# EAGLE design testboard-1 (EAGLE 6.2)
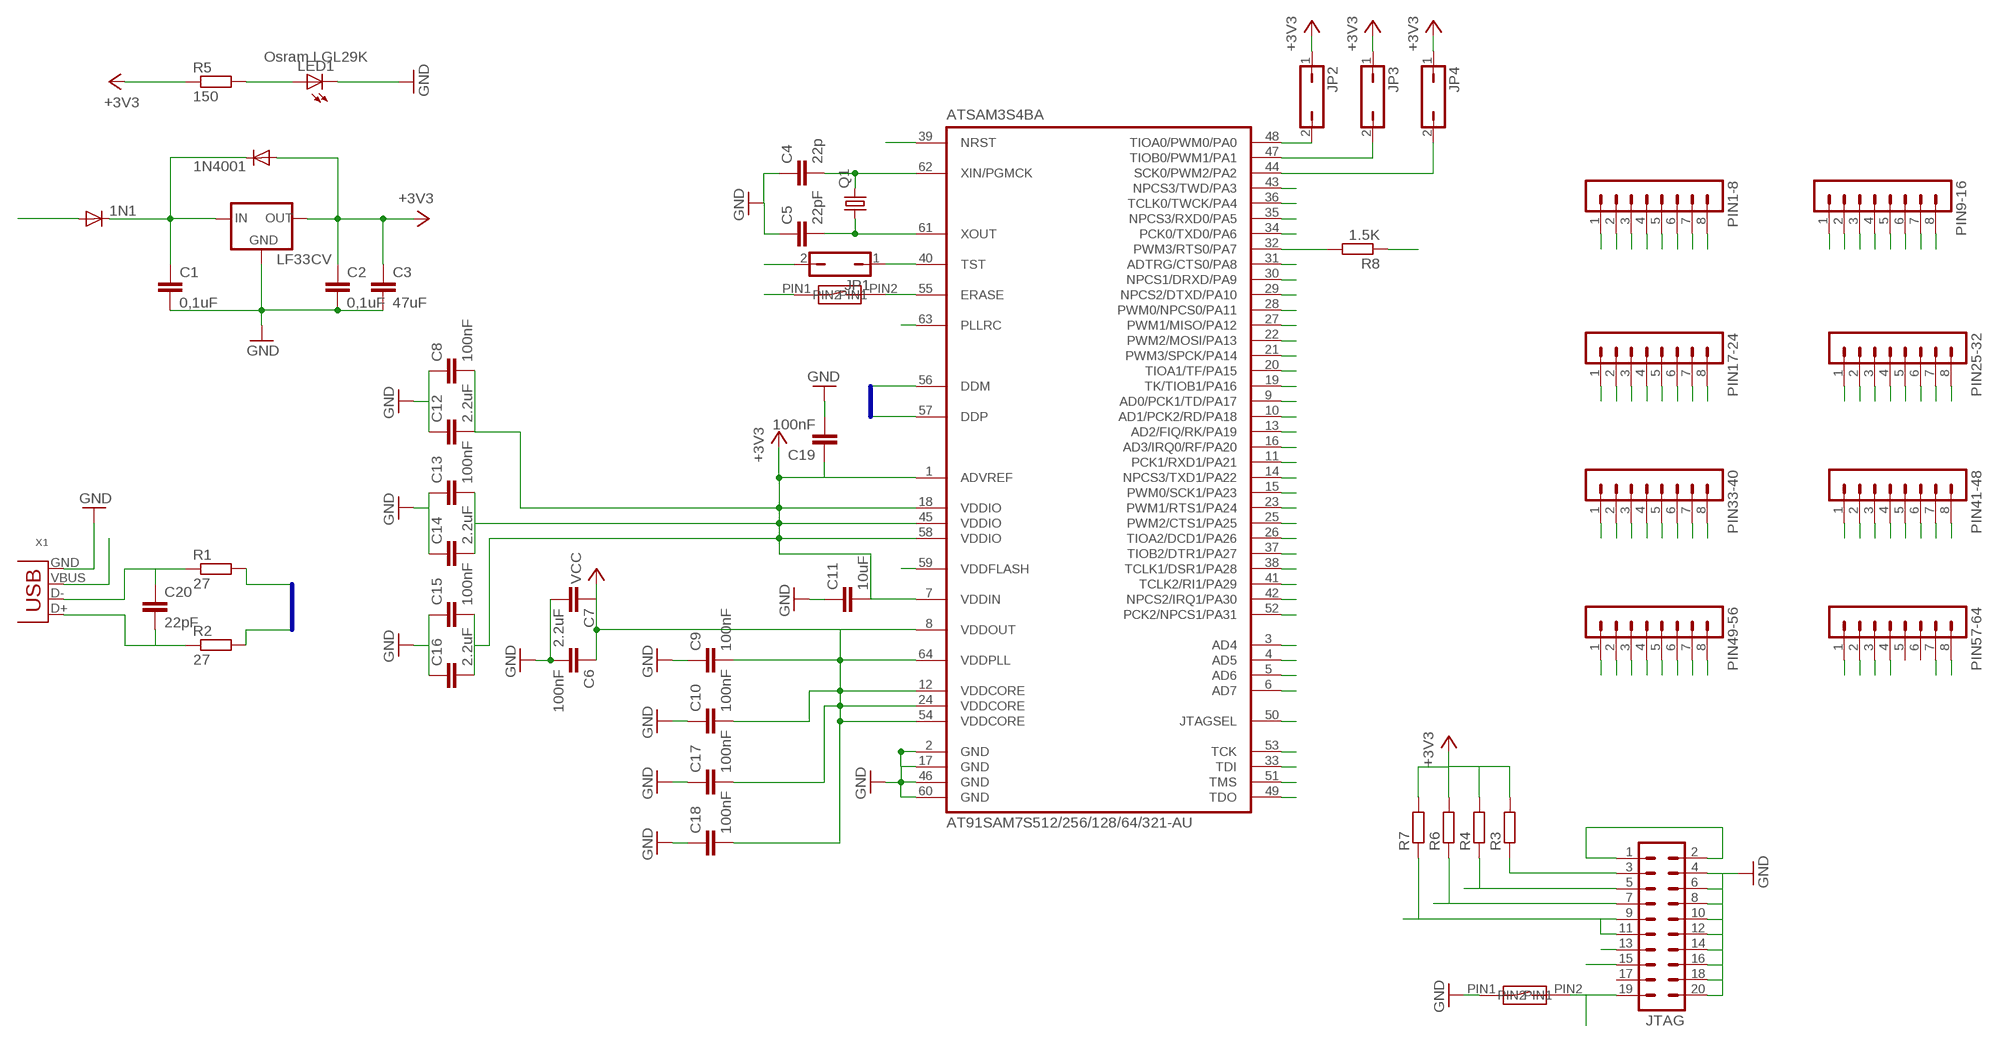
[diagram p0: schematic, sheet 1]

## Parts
1N1  DIODE-MELF-MLL41  [MELF-MLL41]
1N4001  DIODE-MELF-MLL41  [MELF-MLL41]
ATSAM3S4BA  AT91SAM7S512/256/128/64/321-AU  [LQFP64]
C1  0,1uF  C-EUC0805  [C0805]
C2  0,1uF  C-EUC0805  [C0805]
C3  47uF  C-EUC1206  [C1206]
C4  22p  C-EUC0805  [C0805]
C5  22pF  C-EUC0805  [C0805]
C6  100nF  C-EUC0603  [C0603]
C7  2.2uF  C-EUC0603  [C0603]
C8  100nF  C-EUC0603  [C0603]
C9  100nF  C-EUC0603K  [C0603K]
C10  100nF  C-EUC0603  [C0603]
C11  10uF  C-EUC0603  [C0603]
C12  2.2uF  C-EUC0603  [C0603]
C13  100nF  C-EUC0603  [C0603]
C14  2.2uF  C-EUC0603  [C0603]
C15  100nF  C-EUC0603  [C0603]
C16  2.2uF  C-EUC0603  [C0603]
C17  100nF  C-EUC0603  [C0603]
C18  100nF  C-EUC0603  [C0603]
C19  100nF  C-EUC0603  [C0603]
C20  22pF  C-EUC0603  [C0603]
JP1  JP1Q  [JP1]
JP2  JP1Q  [JP1]
JP3  JP1Q  [JP1]
JP4  JP1Q  [JP1]
JTAG  MA10-2  [MA10-2]
LED1  LEDSML0603  [SML0603]
LF33CV  78XXL  [78XXL]
PIN1-8  MA08-1  [MA08-1]
PIN9-16  MA08-1  [MA08-1]
PIN17-24  MA08-1  [MA08-1]
PIN25-32  MA08-1  [MA08-1]
PIN33-40  MA08-1  [MA08-1]
PIN41-48  MA08-1  [MA08-1]
PIN49-56  MA08-1  [MA08-1]
PIN57-64  MA08-1  [MA08-1]
Q1  CRYSTALHC49S  [HC49/S]
R1  27  R-EU_R0603  [R0603]
R2  27  R-EU_R0603  [R0603]
R3  R-EU_R0603  [R0603]
R4  R-EU_R0603  [R0603]
R5  150  R-EU_M0805  [M0805]
R6  R-EU_R0603  [R0603]
R7  R-EU_R0603  [R0603]
R8  1.5K  R-EU_R0603  [R0603]
SWITCH1  SDT21S  [DIL-2]
SWITCH2  SDT21S  [DIL-2]
X1  USB-B-H  [USB-B-H]

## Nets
+3V3: 1N4001.A ATSAM3S4BA.1(ADVREF) ATSAM3S4BA.7(VDDIN) ATSAM3S4BA.18(VDDIO) ATSAM3S4BA.45(VDDIO) ATSAM3S4BA.58(VDDIO) C2.1 C3.1 C8.2 C11.2 C12.2 C13.2 C14.2 C15.2 C16.2 C19.1 JP2.1 JP3.1 JP4.1 LF33CV.OUT R3.2 R4.2 R5.1 R6.2 R7.2
GND: ATSAM3S4BA.2(GND) ATSAM3S4BA.17(GND) ATSAM3S4BA.46(GND) ATSAM3S4BA.60(GND) C1.2 C2.2 C3.2 C4.1 C5.1 C6.2 C7.2 C8.1 C9.1 C10.1 C11.1 C12.1 C13.1 C14.1 C15.1 C16.1 C17.1 C18.1 C19.2 JTAG.4 JTAG.6 JTAG.8 JTAG.10 JTAG.12 JTAG.14 JTAG.16 JTAG.18 JTAG.20 LED1.C LF33CV.GND SWITCH2.PIN1 X1.GND
N$7: C20.1 R1.1 X1.D-
N$13: LED1.A R5.2
N$14: ATSAM3S4BA.59(VDDFLASH)
N$15: ATSAM3S4BA.55(ERASE) SWITCH1.PIN2
N$18: JTAG.3 R3.1
NRST: ATSAM3S4BA.39(NRST) JTAG.15 JTAG.19 SWITCH2.PIN2
PIN1: PIN1-8.1
PIN2: PIN1-8.2
PIN3: ATSAM3S4BA.3(AD4) PIN1-8.3
PIN4: ATSAM3S4BA.4(AD5) PIN1-8.4
PIN5: ATSAM3S4BA.5(AD6) PIN1-8.5
PIN6: ATSAM3S4BA.6(AD7) PIN1-8.6
PIN7: PIN1-8.7
PIN8: PIN1-8.8
PIN9: ATSAM3S4BA.9(AD0/PCK1/TD/PA17) PIN9-16.1
PIN10: ATSAM3S4BA.10(AD1/PCK2/RD/PA18) PIN9-16.2
PIN11: ATSAM3S4BA.11(PCK1/RXD1/PA21) PIN9-16.3
PIN12: PIN9-16.4
PIN13: ATSAM3S4BA.13(AD2/FIQ/RK/PA19) PIN9-16.5
PIN14: ATSAM3S4BA.14(NPCS3/TXD1/PA22) PIN9-16.6
PIN15: ATSAM3S4BA.15(PWM0/SCK1/PA23) PIN9-16.7
PIN16: ATSAM3S4BA.16(AD3/IRQ0/RF/PA20) PIN9-16.8
PIN17: PIN17-24.1
PIN18: PIN17-24.2
PIN19: ATSAM3S4BA.19(TK/TIOB1/PA16) PIN17-24.3
PIN20: ATSAM3S4BA.20(TIOA1/TF/PA15) PIN17-24.4
PIN21: ATSAM3S4BA.21(PWM3/SPCK/PA14) PIN17-24.5
PIN22: ATSAM3S4BA.22(PWM2/MOSI/PA13) PIN17-24.6
PIN23: ATSAM3S4BA.23(PWM1/RTS1/PA24) PIN17-24.7
PIN24: PIN17-24.8
PIN25: ATSAM3S4BA.25(PWM2/CTS1/PA25) PIN25-32.1
PIN26: ATSAM3S4BA.26(TIOA2/DCD1/PA26) PIN25-32.2
PIN27: ATSAM3S4BA.27(PWM1/MISO/PA12) PIN25-32.3
PIN28: ATSAM3S4BA.28(PWM0/NPCS0/PA11) PIN25-32.4
PIN29: ATSAM3S4BA.29(NPCS2/DTXD/PA10) PIN25-32.5
PIN30: ATSAM3S4BA.30(NPCS1/DRXD/PA9) PIN25-32.6
PIN31: ATSAM3S4BA.31(ADTRG/CTS0/PA8) PIN25-32.7
PIN32: ATSAM3S4BA.32(PWM3/RTS0/PA7) PIN25-32.8 R8.2
PIN33: ATSAM3S4BA.33(TDI) JTAG.5 PIN33-40.1 R4.1
PIN34: ATSAM3S4BA.34(PCK0/TXD0/PA6) PIN33-40.2
PIN35: ATSAM3S4BA.35(NPCS3/RXD0/PA5) PIN33-40.3
PIN36: ATSAM3S4BA.36(TCLK0/TWCK/PA4) PIN33-40.4
PIN37: ATSAM3S4BA.37(TIOB2/DTR1/PA27) PIN33-40.5
PIN38: ATSAM3S4BA.38(TCLK1/DSR1/PA28) PIN33-40.6
PIN39: PIN33-40.7
PIN40: ATSAM3S4BA.40(TST) JP1.1 PIN33-40.8
PIN41: ATSAM3S4BA.41(TCLK2/RI1/PA29) PIN41-48.1
PIN42: ATSAM3S4BA.42(NPCS2/IRQ1/PA30) PIN41-48.2
PIN43: ATSAM3S4BA.43(NPCS3/TWD/PA3) PIN41-48.3
PIN44: ATSAM3S4BA.44(SCK0/PWM2/PA2) JP4.2 PIN41-48.4
PIN45: PIN41-48.5
PIN46: PIN41-48.6
PIN47: ATSAM3S4BA.47(TIOB0/PWM1/PA1) JP3.2 PIN41-48.7
PIN48: ATSAM3S4BA.48(TIOA0/PWM0/PA0) JP2.2 PIN41-48.8
PIN49: ATSAM3S4BA.49(TDO) JTAG.13 PIN49-56.1
PIN50: ATSAM3S4BA.50(JTAGSEL) PIN49-56.2
PIN51: ATSAM3S4BA.51(TMS) JTAG.7 PIN49-56.3 R6.1
PIN52: ATSAM3S4BA.52(PCK2/NPCS1/PA31) PIN49-56.4
PIN53: ATSAM3S4BA.53(TCK) JTAG.9 JTAG.11 PIN49-56.5 R7.1
PIN54: PIN49-56.6
PIN55: PIN49-56.7
PIN56: PIN49-56.8
PIN57: PIN57-64.1
PIN58: PIN57-64.2
PIN59: PIN57-64.3
PIN60: PIN57-64.4
PIN61: ATSAM3S4BA.61(XOUT) C5.2 Q1.1
PIN62: ATSAM3S4BA.62(XIN/PGMCK) C4.2 Q1.2
PIN63: ATSAM3S4BA.63(PLLRC) PIN57-64.7
PIN64: PIN57-64.8
USB_5V: 1N1.A X1.VBUS
USB_MINUS: ATSAM3S4BA.56(DDM) R1.2
USB_PLUS: ATSAM3S4BA.57(DDP) R2.2
USB_PLUS_GEHAUSE: C20.2 R2.1 R8.1 X1.D+
VCC18: ATSAM3S4BA.8(VDDOUT) ATSAM3S4BA.12(VDDCORE) ATSAM3S4BA.24(VDDCORE) ATSAM3S4BA.54(VDDCORE) ATSAM3S4BA.64(VDDPLL) C6.1 C7.1 C9.2 C10.2 C17.2 C18.2 JP1.2 JTAG.1 JTAG.2 SWITCH1.PIN1 ; supply symbol labelled VCC
VX: 1N1.C 1N4001.C C1.1 LF33CV.IN
Unconnected: JTAG.17 PIN57-64.5 PIN57-64.6

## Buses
B$2
B$1

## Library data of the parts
1N1 1N4001 = diode:DIODE-: DIODE
ATSAM3S4BA = atmel-arm:AT91SAM7S512/256/128/64/321: AT91SAM7S512/256/128/64/321 ARM7 Processor
C1-C20 = rcl:C-EU: CAPACITOR, European symbol
JP1-JP4 = jumper:JP1Q: JUMPER
JTAG = con-lstb:MA10-2: PIN HEADER; OC_FARNELL: unknown; OC_NEWARK: unknown
LED1 = led:LED: LED; PRODUCT: Osram LGL29K
LF33CV = v-reg:78XXL: VOLTAGE REGULATOR
PIN1-8 PIN9-16 PIN17-24 PIN25-32 PIN33-40 PIN41-48 PIN49-56 PIN57-64 = con-lstb:MA08-1: PIN HEADER; OC_FARNELL: unknown; OC_NEWARK: unknown
Q1 = crystal:CRYSTAL: CRYSTAL; OC_FARNELL: 1667008; OC_NEWARK: unknown
R1-R8 = rcl:R-EU_: RESISTOR, European symbol
SWITCH1 SWITCH2 = reichelt:SDT21S: "Reichelt Switch - 2 DIL"
X1 = con-usb-3:USB: USB Connectors

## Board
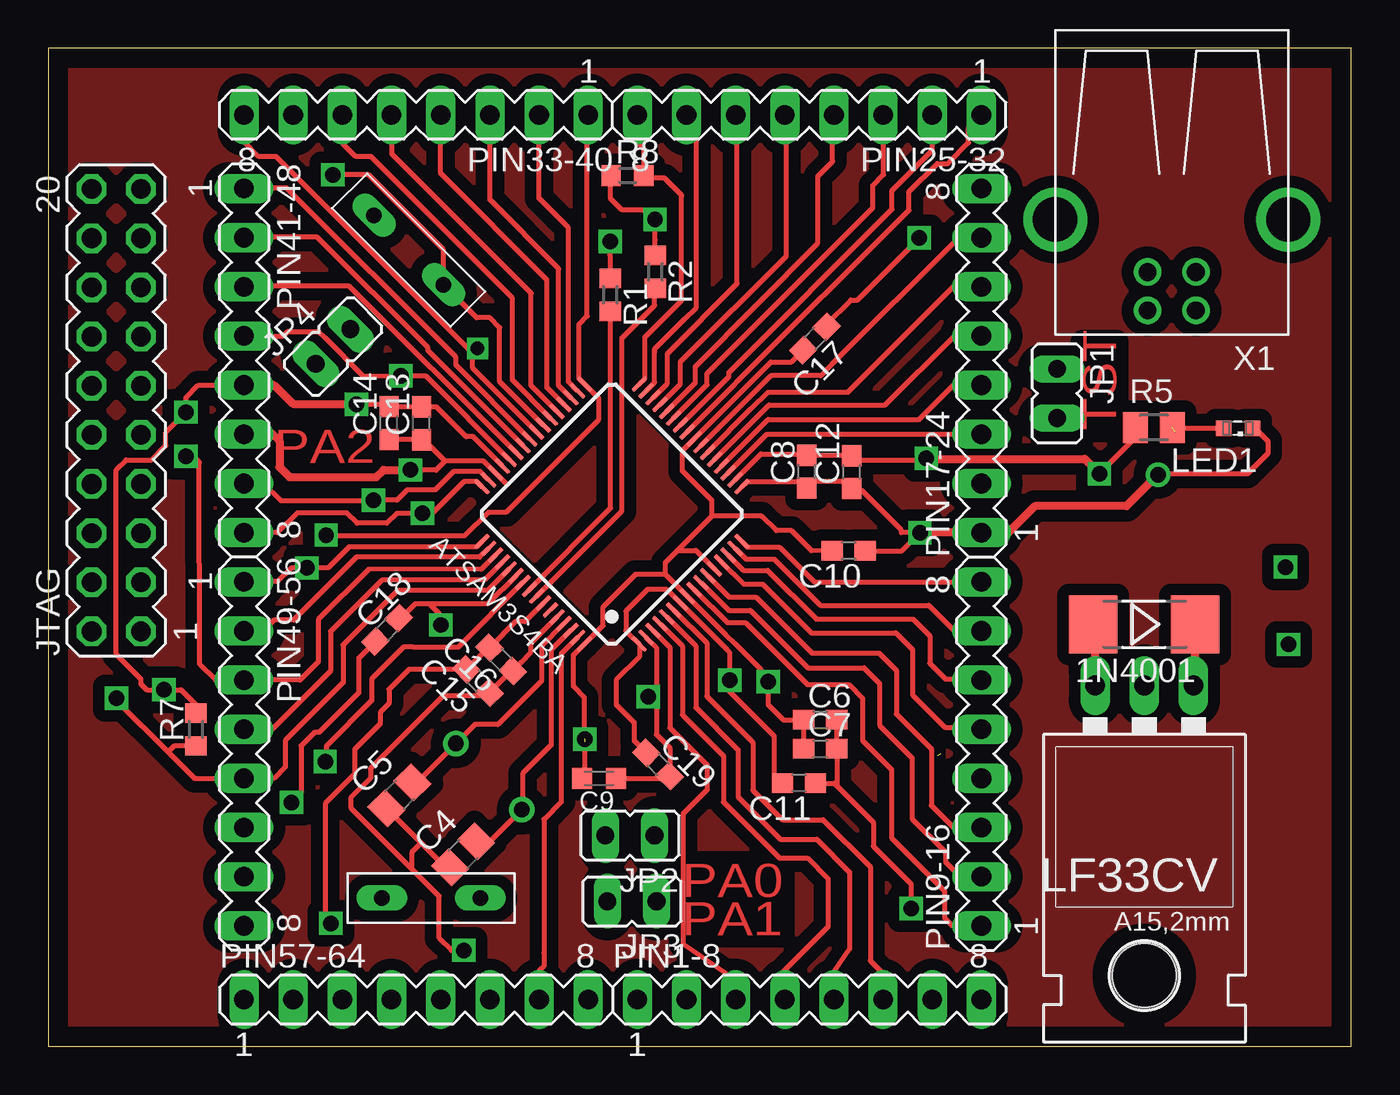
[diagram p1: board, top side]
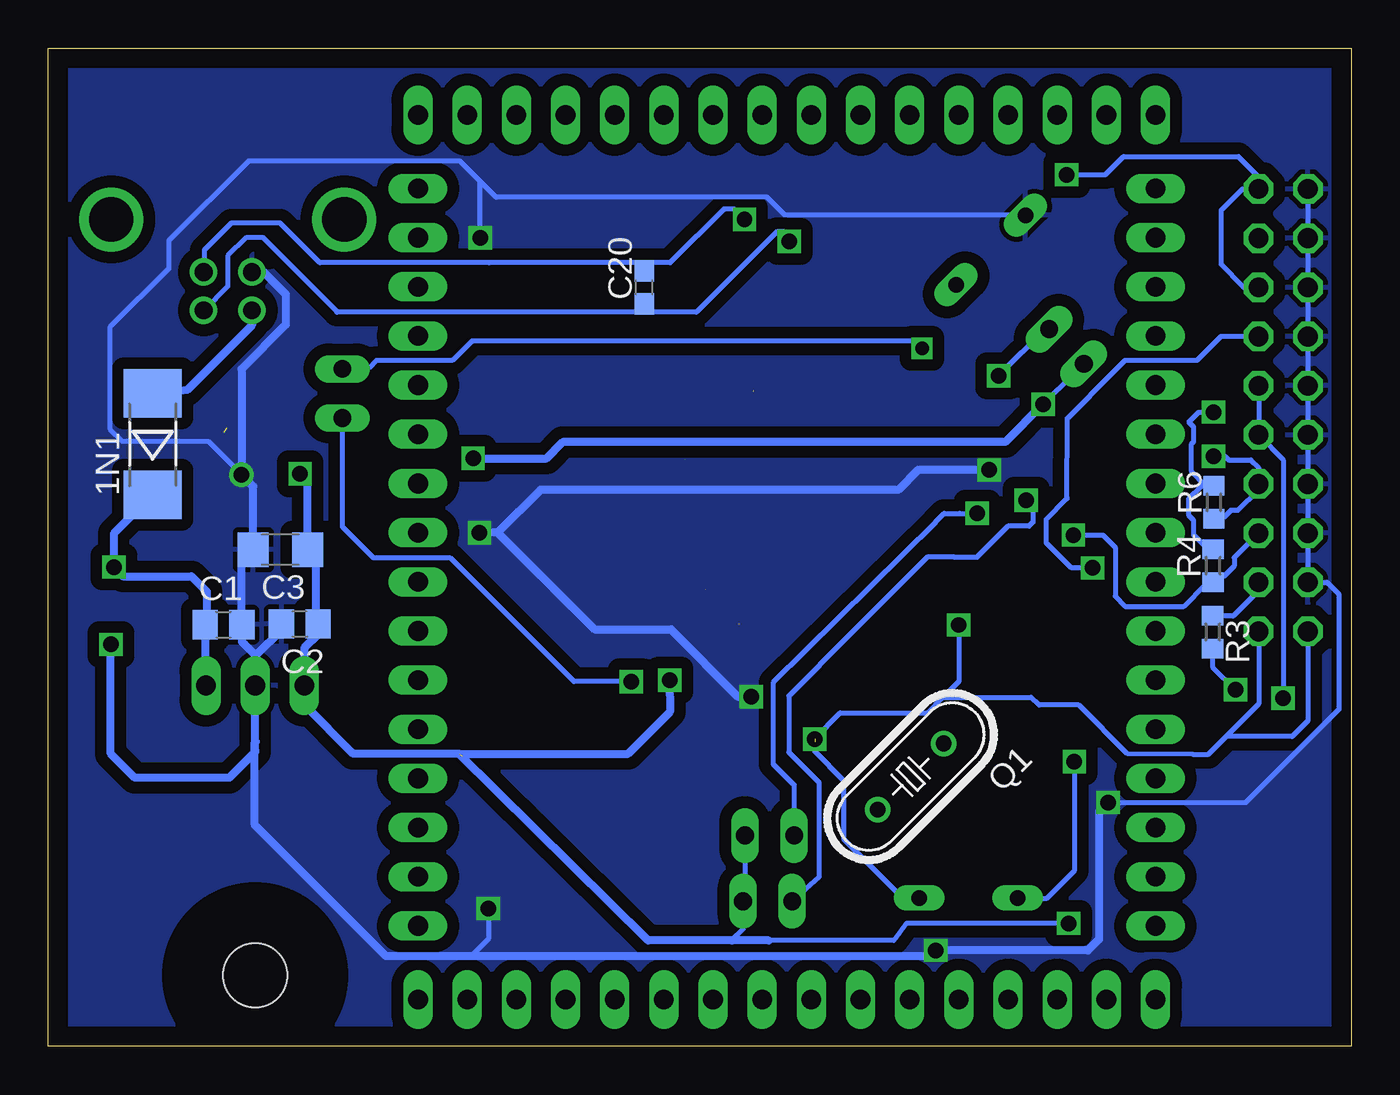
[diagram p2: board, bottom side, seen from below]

Size 67.31 x 51.56 mm. Coordinates in mm from the lower left corner, seen from the top.
Outline: 0,0 67.31,0 67.31,51.56 0,51.56 0,0
Copper layers (1*16): Top 0.035mm / dielectric 1.5mm / Bottom 0.035mm
Design rules "default": minimum track width 10mil, minimum drill 24mil, track to track 8mil, track to pad 8mil, pad to pad 8mil, via to via 8mil, smd to smd 8mil, copper to edge 40mil, drill to drill 8mil, minimum pad ring 10mil, minimum via ring 8mil, stop-mask expansion 4mil, vias tented up to drill 0mil, thermal gap 10mil

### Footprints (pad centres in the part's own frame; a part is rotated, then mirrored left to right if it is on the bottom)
MELF-MLL41 = smd 2.5 x 3: A 2.625,0; C -2.625,0
LQFP64 = smd 0.25 x 1: 1 -3.75,-5.75; 2 -3.25,-5.75; 3 -2.75,-5.75; 4 -2.25,-5.75; 5 -1.75,-5.75; 6 -1.25,-5.75; 7 -0.75,-5.75; 8 -0.25,-5.75; 9 0.25,-5.75; 10 0.75,-5.75; 11 1.25,-5.75; 12 1.75,-5.75; 13 2.25,-5.75; 14 2.75,-5.75; 15 3.25,-5.75; 16 3.75,-5.75; 33 3.75,5.75; 34 3.25,5.75; 35 2.75,5.75; 36 2.25,5.75; 37 1.75,5.75; 38 1.25,5.75; 39 0.75,5.75; 40 0.25,5.75; 41 -0.25,5.75; 42 -0.75,5.75; 43 -1.25,5.75; 44 -1.75,5.75; 45 -2.25,5.75; 46 -2.75,5.75; 47 -3.25,5.75; 48 -3.75,5.75 | smd 1 x 0.25: 17 5.75,-3.75; 18 5.75,-3.25; 19 5.75,-2.75; 20 5.75,-2.25; 21 5.75,-1.75; 22 5.75,-1.25; 23 5.75,-0.75; 24 5.75,-0.25; 25 5.75,0.25; 26 5.75,0.75; 27 5.75,1.25; 28 5.75,1.75; 29 5.75,2.25; 30 5.75,2.75; 31 5.75,3.25; 32 5.75,3.75; 49 -5.75,3.75; 50 -5.75,3.25; 51 -5.75,2.75; 52 -5.75,2.25; 53 -5.75,1.75; 54 -5.75,1.25; 55 -5.75,0.75; 56 -5.75,0.25; 57 -5.75,-0.25; 58 -5.75,-0.75; 59 -5.75,-1.25; 60 -5.75,-1.75; 61 -5.75,-2.25; 62 -5.75,-2.75; 63 -5.75,-3.25; 64 -5.75,-3.75
C0805 = smd 1.3 x 1.5: 1 -0.95,0; 2 0.95,0
C1206 = smd 1.6 x 1.8: 1 -1.4,0; 2 1.4,0
C0603 = smd 1.1 x 1: 1 -0.85,0; 2 0.85,0
C0603K = smd 1.05 x 1.08: 1 -0.875,0; 2 0.875,0
JP1 = drill 0.914 long: 1 0,-1.27; 2 0,1.27
MA10-2 = drill 1.016 octagon: 1 -11.43,-1.27; 2 -11.43,1.27; 3 -8.89,-1.27; 4 -8.89,1.27; 5 -6.35,-1.27; 6 -6.35,1.27; 7 -3.81,-1.27; 8 -3.81,1.27; 9 -1.27,-1.27; 10 -1.27,1.27; 11 1.27,-1.27; 12 1.27,1.27; 13 3.81,-1.27; 14 3.81,1.27; 15 6.35,-1.27; 16 6.35,1.27; 17 8.89,-1.27; 18 8.89,1.27; 19 11.43,-1.27; 20 11.43,1.27
SML0603 = smd 0.8 x 0.8: A 0.75,0; C -0.75,0
78XXL = drill 1.016 long: GND 0,-3.81; IN -2.54,-3.81; OUT 2.54,-3.81 | hole 3.302: 0,11.176
MA08-1 = drill 1.016 long: 1 -8.89,0; 2 -6.35,0; 3 -3.81,0; 4 -1.27,0; 5 1.27,0; 6 3.81,0; 7 6.35,0; 8 8.89,0
HC49/S = drill 0.813: 1 -2.413,0; 2 2.413,0
R0603 = smd 1 x 1.1: 1 -0.85,0; 2 0.85,0
M0805 = smd 1.3 x 1.6: 1 -0.95,0; 2 0.95,0
DIL-2 = drill 0.8 long: PIN1 -2.54,0; PIN2 2.54,0
USB-B-H = drill 0.914: D+ 0,1.25; D- 1.981,1.25; GND 0,-1.25; VBUS 1.981,-1.25 | drill 2.286: P$1 -2.718,-6.02; P$2 -2.718,6.02

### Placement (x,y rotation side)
1N1  61.93,31.11 90 bottom
1N4001  56.61,21.8 180 top
ATSAM3S4BA  29.12,27.5 45 top
C1  58.26,21.78 0 bottom
C2  54.32,21.82 180 bottom
C3  55.32,25.66 180 bottom
C4  21.43,9.91 45 top
C5  18.14,12.97 45 top
C6  39.88,16.87 0 top
C7  39.88,15.37 0 top
C8  39.19,29.69 90 top
C9  28.45,13.84 180 top
C10  41.35,25.6 180 top
C11  38.78,13.59 180 top
C12  41.5,29.67 90 top
C13  19.28,32.19 90 top
C14  17.6,32.2 90 top
C15  22.2,18.87 135 top
C16  23.39,19.99 135 top
C17  39.6,36.57 225 top
C18  17.5,21.52 45 top
C19  31.5,14.55 315 top
C20  36.53,39.22 90 bottom
JP1  52.12,33.73 180 top
JP2  30.05,10.89 90 top
JP3  30.15,7.49 90 top
JP4  14.71,36.16 315 top
JTAG  3.51,32.86 90 top
LED1  61.46,31.94 180 top
LF33CV  56.63,14.83 180 top
PIN1-8  39.32,2.41 0 top
PIN9-16  48.21,15.11 90 top
PIN17-24  48.21,35.43 90 top
PIN25-32  39.32,48.13 180 top
PIN33-40  19,48.13 180 top
PIN41-48  10.11,35.43 270 top
PIN49-56  10.11,15.11 270 top
PIN57-64  19,2.41 0 top
Q1  22.76,13.94 225 bottom
R1  29.03,38.82 270 top
R2  31.35,40.01 270 top
R3  7.16,21.4 270 bottom
R4  7.14,24.83 90 bottom
R5  57.12,31.97 0 top
R6  7.09,28.11 90 bottom
R7  7.62,16.37 90 top
R8  29.92,44.98 0 top
SWITCH1  19.77,7.66 180 top
SWITCH2  18.62,41.15 315 top
X1  58.04,40 270 top

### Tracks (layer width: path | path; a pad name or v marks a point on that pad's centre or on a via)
+3V3  (via drill 0.8)  (1 unrouted)
  Top 0.254: R5.1 56.16,31.45 v54.3,29.59 | C11.2 37.49,14.04 37.49,16.03 35.22,18.3 35.22,18.96 v35.21,18.91 35.2,18.97 35.2,20.34 35.08,20.47 35.08,20.48 ATSAM3S4BA.7 31.93,23.62 30.99,23.62 29.84,22.48 29.84,21.46 29.97,21.34 ATSAM3S4BA.1 30.53,20.12 29.34,18.92 29.34,17.65 30.28,16.71 30.28,15.77 C19.1 | 10.74,34.16 7.75,34.16 7.11,33.53 v7.11,32.77 6.07,31.73 6.07,31.04 5.33,30.3 4.01,30.3 3.5,29.79 3.5,20.24 4.78,18.97 4.78,18.72 5.08,18.41 v5.97,18.41 6.86,18.41 7.62,17.65 R7.2 | ATSAM3S4BA.18 35.51,29.29 36.82,30.6 39.13,30.6 C8.2 | ATSAM3S4BA.45 23.44,29.99 21.95,31.49 21.59,31.49 20.07,33.02 19.3,33.02 C13.2 | ATSAM3S4BA.58 25.56,22.88 24.63,21.94 24.14,21.94 C16.2 22.71,20.59 C15.2 18.64,19.47 17.6,18.44 17.6,17.7 17.14,17.25 17.14,16.66 15.82,15.34 15.82,14.07 14.3,12.55 14.3,6.66 v14.61,6.35 | 19.43,32.89 C13.2 | 17.48,32.91 C14.2 | C13.2 17.61,33.04 C14.2 | v15.92,33.17 17.48,33.17 C14.2 | 38.87,30.6 C8.2 | C8.2 41.48,30.54 C12.2 41.48,30.29 45.28,30.29 v45.36,30.38
  Top 0.406: 10.74,34.16 11.66,34.16 12.65,33.2 v15.92,33.17 | LF33CV.OUT 54.09,21.71 1N4001.A | v54.3,29.59 53.54,30.35 45.8,30.35 v45.36,30.38
  Bottom 0.254: 7.47,20.17 R3.2 7.16,19.61 v5.97,18.41 | v7.11,32.77 7.87,32.77 8.38,32.26 8.13,32 8.13,31.24 8.26,31.11 8.26,29.72 7.5,28.96 R6.2 7.22,28.96 7.75,28.96 8.38,28.32 8.38,27.43 8.13,27.18 8.13,26.42 7.4,25.68 R4.2 | v14.61,6.35 22.99,6.35 23.62,5.46 30.1,5.46 | v35.21,18.91 35.23,18.97 35.27,18.93 | JP4.1 13.81,35.21 v15.92,33.17 | JP2.1 31.32,7.59 JP3.1 31.42,6.04 32,5.46
  Bottom 0.406: v54.3,29.59 53.92,29.2 C3.1 53.47,25.2 53.47,21.82 C2.1 53.37,21.29 54.09,20.57 LF33CV.OUT 54.1,18.63 54.1,17.65 51.56,15.11 46.1,15.11 | 46.1,15.11 36.32,5.46 32,5.46 30.1,5.46 | v45.36,30.38 41.58,30.38 40.74,31.21 17.87,31.22 v15.92,33.17 | v35.21,18.91 35.2,17.28 37.37,15.11 46.1,15.11 | 45.94,14.99 45.96,14.97
GND  (via drill 0.8, 0.8 pad 1.27)
  Top 0.254: ATSAM3S4BA.17 35.84,28.92 36.11,29.19 38.84,29.19 C8.1 39.26,28.84 39.62,29.21 41.11,29.21 C12.1 | 20.5,30.23 22.5,30.23 22.61,30.12 22.62,30.11 ATSAM3S4BA.46 23.65,29.08 | 20.5,30.23 20.04,29.77 v18.69,29.78 18.2,29.78 | ATSAM3S4BA.60 26.27,22.18 24.91,20.82 24.91,20.34 24.38,19.81 24.38,19.78 C16.1 23.91,19.39 C15.1 22.8,18.1 20.38,18.1 16.64,14.35 16.64,13.84 15.62,12.83 15.62,12.32 18.8,9.14 | LED1.C 62.33,31.95 63.02,31.27 63.02,30.63 61.95,29.57 57.35,29.56 v57.33,29.54 | C17.1 40.2,37.32 41.46,38.56 41.81,38.56 v45,41.76 | C18.1 16.05,20.07 16.05,18.28 14,16.23 13.76,16.23 13.06,15.52 13.06,13.11 v12.55,12.6 | C6.2 C7.2 40.74,15.35 40.74,13.46 | C11.1 40.61,13.59 40.74,13.46 | 40.74,13.46 42.62,11.58 42.62,10.34 44.58,8.38 v44.58,7.11 | v21.46,4.95 20.83,4.95 20.19,5.59 20.19,7.75 18.8,9.14 | ATSAM3S4BA.2 31.42,20.6 31.42,18.49 | 31.42,18.49 31.42,16.1 32.11,15.42 32.11,13.96 C19.2 31.98,13.84 C9.1 | v30.99,18.06 31.42,18.49 | C10.1 44.09,25.6 v45.03,26.54 44.07,26.54 44.07,26.67 42.04,28.7 41.62,28.7 C12.1 | C14.1 17.61,31.34 C13.1 19.39,31.34 20.5,30.23 | 41.51,28.57 C12.1 | 41.48,28.59 C12.1 | C4.1 20.52,9.24 19.26,10.5 | 19.26,10.5 C5.1 | 18.8,9.14 18.8,10.03 19.26,10.5
  Top 0.406: v57.33,29.54 55.7,27.91 50.98,27.91 49.61,26.54 v45.03,26.54 44.93,26.54
  Bottom 0.254: 56.59,15.19 56.59,15.75 56.59,18.61 LF33CV.GND | SWITCH2.PIN1 17.37,42.95 29.26,42.95 30.18,43.87 44.17,43.87 45,44.69 | 45,44.69 46.05,45.74 56.97,45.74 61.09,41.63 61.09,40.18 64.14,37.16 64.14,31.9 63.5,31.27 59.05,31.27 v57.33,29.54 | JTAG.20 JTAG.18 JTAG.16 JTAG.14 JTAG.12 JTAG.10 JTAG.8 JTAG.6 JTAG.4 1.24,23.97 0.64,23.37 0.64,17.4 5.44,12.6 v12.55,12.6 | v44.58,7.11 44.58,5.54 45.47,4.65 | v45,41.76 45,44.69
  Bottom 0.406: X1.GND 56.19,40 55.04,38.86 55.04,37.28 57.33,35 v57.33,29.54 56.72,28.93 C3.2 57.31,25.06 C1.2 57.31,20.91 56.59,20.19 | v30.99,18.06 31.67,18.06 35.13,21.54 39.09,21.54 44.09,26.54 | 56.59,20.19 56.59,18.68 LF33CV.GND | C2.2 55.27,21.51 56.59,20.19 | v18.69,29.78 22.38,29.78 23.4,28.75 25.3,28.75 39.27,28.75 41.88,28.75 44.09,26.54 | v12.55,12.6 13.03,12.12 13.03,5.51 13.59,4.95 v21.46,4.95 21.77,4.65 45.47,4.65 49.86,4.65 56.64,11.43 56.64,15.7 56.59,15.75 | 44.09,26.54 v45.03,26.54
  pour Bottom (isolate 0.61): 0,-0.13 67.44,-0.13 67.44,51.69 -0.13,51.69 -0.13,0
N$2  (via drill 0.8 pad 1.02)
  other vias: 64.08,20.76
N$3
  Bottom 0.406: 56.62,15.21 57.96,13.87 62.84,13.87 64.08,15.11 64.08,20.75
N$4
  Bottom 0.406: 56.62,15.26 56.62,18.62
N$6
  pour Top (isolate 0.61): 0,0 67.39,0 67.39,51.51 -0.19,51.51 -0.19,0.25
N$7  (via drill 0.8)
  Top 0.254: R1.1 29.04,40.81 29.03,40.82 v29.03,41.58
  Bottom 0.254: X1.D- 58.04,39.27 58.04,40.84 57.1,41.78 56.21,41.78 52.4,37.97 52.4,37.92 36.52,37.92 | v29.03,41.58 29.03,41.83 29.29,42.09 29.67,42.09 33.83,37.92 36.52,37.92 | C20.1 36.52,37.92
N$9
  Top 0.406: 10.2,31.65 10.21,31.63 11.56,31.63 11.94,31.27 11.94,29.92 12.45,29.41 16.94,29.41 17.32,29.78 18.73,29.78 18.73,29.77
N$13  (1 unrouted)
  Top 0.254: 58.23,31.74 58.71,31.94 LED1.A
N$15  (via drill 0.8)
  Top 0.254: ATSAM3S4BA.55 21.19,20.63 18.85,20.62 18.36,20.62 16.71,18.97 16.71,17.86 14.35,15.49 14.35,14.76 v14.3,14.71
  Bottom 0.254: v14.3,14.71 14.3,9.07 15.75,7.62 17.2,7.62 SWITCH1.PIN2
N$18
  Bottom 0.254: JTAG.3 4.78,23.54 6.1,22.23 7.14,22.23 R3.1
NRST  (via drill 0.8)
  Top 0.254: ATSAM3S4BA.39 25.57,32.1 23.32,34.34 23.32,37.13 22.81,37.64 22.12,37.64 SWITCH2.PIN2 20.41,41.16 16.54,45.03 v14.71,45.03
  Bottom 0.254: v14.71,45.03 12.7,45.03 11.76,45.97 5.82,45.97 4.83,44.96 4.78,44.91 JTAG.19 5.62,44.29 6.73,43.18 6.73,40.4 5.59,39.24 5.56,39.21 JTAG.15
PIN3
  Top 0.254: ATSAM3S4BA.3 31.28,21.44 32.11,20.61 32.11,16.45 34.04,14.53 34.04,13.25 32.79,12.01 32.79,5.28 35.51,3.43 PIN1-8.3
PIN4  (1 unrouted)
  Top 0.254: 31.63,21.81 32.76,20.67 32.76,17.12 34.87,15.01 34.87,12.62 37.77,9.73 39.22,9.73 40.28,8.66 40.28,6.17 37.97,3.86 37.97,2.49 PIN1-8.4
PIN5
  Top 0.254: ATSAM3S4BA.5 31.97,22.17 33.45,20.68 33.45,17.5 35.64,15.32 35.64,12.88 37.82,10.69 39.7,10.69 41.4,8.99 41.4,5.03 40.59,3.86 PIN1-8.5
PIN6
  Top 0.254: ATSAM3S4BA.6 34.02,20.83 34.02,18.08 36.4,15.7 36.4,13.23 37.92,11.71 40.03,11.71 42.47,9.27 42.47,4.42 43.13,3.76 PIN1-8.6
PIN9  (1 unrouted)
  Top 0.254: ATSAM3S4BA.9 35.08,21.89 36.02,21.89 39.22,18.69 41.35,18.69 42.06,17.98 42.06,15.8 43.56,14.3 43.56,10.77 46.3,8.02 46.3,6.63 46.71,6.22 PIN9-16.1
PIN10
  Top 0.254: ATSAM3S4BA.10 35.15,22.53 36.27,22.53 39.24,19.55 42.14,19.55 42.95,18.74 42.95,16.58 44.63,14.91 44.63,11.76 46.35,10.03 46.35,9.53 47.12,8.76 PIN9-16.2 48.18,8.79
PIN11
  Top 0.254: ATSAM3S4BA.11 35.17,23.21 36.55,23.21 39.45,20.32 42.93,20.32 43.81,19.43 43.81,17.17 45.62,15.36 45.62,12.44 46.76,11.3 PIN9-16.3
PIN13
  Top 0.254: ATSAM3S4BA.13 34.79,25 35.93,23.87 36.91,23.87 39.42,21.36 43.79,21.36 44.65,20.5 44.65,18.16 46.33,16.48 48.11,16.48 PIN9-16.5
PIN14
  Top 0.254: ATSAM3S4BA.14 35.92,24.59 37.16,24.59 39.67,22.07 44.68,22.07 45.54,21.21 45.54,19.78 46.35,18.97 48.16,18.97 PIN9-16.6
PIN15
  Top 0.254: ATSAM3S4BA.15 35.49,25.71 36.05,25.17 37.5,25.17 39.9,22.78 45.49,22.78 46.81,21.46 PIN9-16.7
PIN16
  Top 0.254: ATSAM3S4BA.16 36.12,25.8 37.77,25.8 39.57,24 PIN9-16.8
PIN19
  Top 0.254: ATSAM3S4BA.19 35.13,29.63 37.13,31.62 PIN17-24.3
PIN20
  Top 0.254: ATSAM3S4BA.20 37.19,32.39 44.98,32.39 46.76,34.16 PIN17-24.4
PIN21  (1 unrouted)
  Top 0.254: PIN17-24.5 46.8,36.7 43.24,33.13 37.23,33.14 ATSAM3S4BA.21 | ATSAM3S4BA.21
PIN22
  Top 0.254: ATSAM3S4BA.22 34.09,30.71 36.31,32.94 37.18,33.8 41.32,33.8 46.76,39.24 PIN17-24.6
PIN23
  Top 0.254: ATSAM3S4BA.23 33.73,31.05 37.33,34.65 39.91,34.65 40.47,35.22 47.01,41.76 48.18,41.76 PIN17-24.7
PIN25
  Top 0.254: ATSAM3S4BA.25 35.48,34.22 35.62,34.36 44.48,43.19 44.48,44.17 45.92,45.62 46.48,45.62 47.55,46.68 47.55,47.47 PIN25-32.1
PIN26
  Top 0.254: ATSAM3S4BA.26 35.15,34.59 35.15,34.82 43.59,43.25 43.59,44.22 45.67,46.3 PIN25-32.2
PIN27
  Top 0.254: ATSAM3S4BA.27 34.04,34.19 34.04,34.77 42.6,43.33 42.6,44.47 43.16,45.03 43.16,48.1 PIN25-32.3
PIN28
  Top 0.254: ATSAM3S4BA.28 31.96,32.81 33.43,34.29 33.43,35.13 39.75,41.5 39.75,44.95 40.51,45.72 40.51,48.05 PIN25-32.4
PIN29
  Top 0.254: ATSAM3S4BA.29 31.6,33.16 32.66,34.22 32.66,35.38 38.12,40.81 38.12,48.05 PIN25-32.5
PIN30
  Top 0.254: ATSAM3S4BA.30 31.26,33.52 31.98,34.25 31.98,35.79 35.59,39.42 35.59,48.05 PIN25-32.6
PIN31  (1 unrouted)
  Top 0.254: PIN25-32.7 33.48,47.62 33.48,38.17 32.89,37.59 31.32,36.01 31.33,35.88 31.33,34.3 31.29,34.26 30.9,33.88
PIN32
  Top 0.254: ATSAM3S4BA.32 30.55,34.23 30.82,34.51 30.82,36.64 32.72,38.53 32.72,43.97 31.83,44.86 30.9,44.86 R8.2 30.77,46.37 30.43,46.71 PIN25-32.8
PIN33  (via drill 0.8)
  Top 0.254: PIN33-40.1 27.84,48.08 27.84,37.72 27.41,37.29 27.41,34.5 27.69,34.22 ATSAM3S4BA.33 27.71,34.21 28.42,33.5 28.42,32.36 23.65,27.58 22.73,27.58 21.51,26.36 14.4,26.36 v14.35,26.42
  Bottom 0.254: JTAG.5 6.04,25.25 6.04,24.82 6.6,24.26 7.25,24.26 R4.1 7.52,23.85 8.64,22.73 11.68,22.73 12.19,23.24 12.19,25.78 12.83,26.42 v14.35,26.42
PIN34
  Top 0.254: ATSAM3S4BA.34 26.87,34.34 26.87,42.29 25.35,43.81 PIN33-40.2
PIN35
  Top 0.254: ATSAM3S4BA.35 26.36,34.13 26.36,40.18 22.81,43.74 PIN33-40.3
PIN36
  Top 0.254: ATSAM3S4BA.36 25.76,34.03 25.76,39.6 20.27,45.11 PIN33-40.4
PIN37
  Top 0.254: ATSAM3S4BA.37 24.94,34.13 24.94,38.91 17.75,46.1 17.75,48.1 PIN33-40.5
PIN38
  Top 0.254: ATSAM3S4BA.38 25.92,32.46 23.98,34.41 23.98,38.66 16.66,45.97 15.88,45.97 15.24,46.61 15.24,48.08 PIN33-40.6
PIN40  (via drill 0.7)
  Top 0.254: 21.92,35.81 11.76,45.97 10.87,45.97 10.11,46.73 PIN33-40.8 | ATSAM3S4BA.40 21.92,35.05 21.92,35.81 | 21.92,35.81 v22.17,36.06
  Bottom 0.254: v22.17,36.06 22.55,36.45 45.41,36.45 46.43,35.43 50.37,35.43 50.75,35.05 52.07,35.05 JP1.1
PIN41
  Top 0.254: ATSAM3S4BA.41 24.85,31.41 21.06,35.2 21.06,35.61 12.32,44.35 10.13,44.35 PIN41-48.1
PIN42
  Top 0.254: ATSAM3S4BA.42 24.5,31.05 19.61,35.95 19.61,36.09 13.89,41.81 10.13,41.81 PIN41-48.2
PIN43
  Top 0.254: ATSAM3S4BA.43 24.14,30.71 15.54,39.27 10.13,39.27 PIN41-48.3
PIN44  (via drill 0.8)
  Top 0.254: ATSAM3S4BA.44 19.61,34.52 19.48,34.64 v18.21,34.64 16.27,34.64 16.22,34.68 14.29,36.61 13.97,36.93 12.37,36.93 12.13,36.7 PIN41-48.4
  Bottom 0.254: JP4.2 15.8,37.05 v18.21,34.64
PIN47  (via drill 0.8)
  Top 0.254: ATSAM3S4BA.47 22.34,29.69 20.93,29.69 19.99,28.75 18.54,28.75 18.01,28.22 v16.79,28.22 16.76,28.19 12.01,28.19 11.12,29.08 PIN41-48.7
  Bottom 0.254: JP3.2 27.51,8.73 27.51,13.64 29.06,15.19 29.06,18.11 25.88,21.28 21.89,25.27 20.5,25.28 19.33,25.28 17.73,26.87 16.64,26.87 16.43,27.08 16.43,27.89 16.76,28.22 v16.79,28.22
PIN48  (via drill 0.8)
  Top 0.254: 22.12,29.18 22.13,29.18 ATSAM3S4BA.48 22.36,28.94 22.12,29.18 | 22.12,29.18 21.49,29.18 19.84,27.53 v19.33,27.53 18.01,27.53 17.5,27.03 15.95,27.03 15.42,27.56 12.88,27.56 11.84,26.54 PIN41-48.8
  Bottom 0.254: JP2.2 28.78,13.51 29.87,14.58 29.87,18.79 21.49,27.07 21.49,27.08 21.03,27.53 20.22,27.53 v19.33,27.53
PIN49  (via drill 0.8)
  Top 0.254: ATSAM3S4BA.49 22.11,25.8 15.54,25.8 14.45,24.71 v13.36,24.71 12.57,24.71 11.84,24 PIN49-56.1
  Bottom 0.254: JTAG.13 6.73,36.67 7.97,35.43 11.68,35.44 12.31,34.8 14.67,32.44 14.68,28.34 14.68,28.3 15.75,27.23 15.75,26.01 14.45,24.71 v13.36,24.71
PIN50
  Top 0.254: ATSAM3S4BA.50 22.29,25.27 15.92,25.27 12.68,22.02 11.66,22.02 11.18,21.54 10.19,21.54 PIN49-56.2
PIN51  (via drill 0.8)
  Top 0.254: ATSAM3S4BA.51 23.09,25.36 22.38,24.65 16.54,24.64 13.95,22.05 13.95,19.86 13.01,18.92 PIN49-56.3 8.64,18.92 7.82,19.74 7.8,30.18 7.49,30.48 v7.11,30.48
  Bottom 0.254: v7.11,30.48 6.5,30.48 6.33,30.3 5.18,30.3 4.78,29.9 4.78,29.69 JTAG.7 4.78,28.75 5.84,27.69 6.22,27.69 6.6,27.3 7.17,27.3 R6.1
PIN52
  Top 0.254: ATSAM3S4BA.52 22.53,24.09 17.25,24.09 14.58,21.43 14.58,19.4 11.56,16.38 PIN49-56.4
PIN53  (via drill 0.8)
  Top 0.254: ATSAM3S4BA.53 22.7,23.56 18.04,23.56 15.22,20.74 15.23,18.79 12.24,15.8 12.24,14.43 11.66,13.84 PIN49-56.5 8.64,13.84 7.55,13.84 6.18,15.2 | v3.51,17.98 3.51,17.88 6.18,15.2 | R7.1 6.5,15.52 6.18,15.2
  Bottom 0.254: JTAG.11 JTAG.9 3.51,30.3 3.5,20.93 3.5,19.36 v3.51,17.98
PIN61
  Top 0.254: ATSAM3S4BA.61 25.47,20.66 25.47,18.87 23.23,16.63 22.04,16.63 Q1.1 19.05,13.64 C5.2
PIN62
  Top 0.254: ATSAM3S4BA.62 25.98,20.47 25.98,19.68 25.98,16.15 25.98,15.56 24.51,14.1 24.51,12.28 Q1.2 22.82,10.59 C4.2
PIN63
  Top 0.254: ATSAM3S4BA.63 27.33,21.11 26.49,20.27 26.49,19.22 26.5,12.62 25.61,11.73 25.6,4.85 25.6,4.14 25.35,3.89 PIN57-64.7
USB_5V
  Bottom 0.406: X1.VBUS 56.79,37.27 60.15,33.91 61.42,33.74 1N1.A
USB_MINUS
  Top 0.254: ATSAM3S4BA.56 24.84,23.57 24.85,23.59 24.85,23.6 29.06,27.81 29.06,38.33 R1.2 29.03,38.35
USB_PLUS
  Top 0.254: ATSAM3S4BA.57 28.39,26.42 28.39,26.43 29.63,27.67 29.63,36.59 29.64,36.6 31.32,38.28 31.32,39.38 R2.2
USB_PLUS_GEHAUSE  (via drill 0.8)
  Top 0.254: R2.1 31.35,41.67 v31.34,42.72 31.27,42.72 30.79,43.2 29.64,43.2 29.06,43.79 29.06,44.97 R8.1
  Bottom 0.254: X1.D+ 59.26,40.03 59.26,41.15 57.86,42.54 55.35,42.54 53.29,40.48 44.53,40.49 36.52,40.49 | v31.34,42.72 31.88,43.26 32.41,43.26 35.18,40.49 36.52,40.49 | C20.2 36.52,40.49
VCC18  (via drill 0.8)  (1 unrouted)
  Top 0.254: ATSAM3S4BA.64 27.12,20.19 27.11,20.19 | ATSAM3S4BA.64 27.11,20.19 | C17.2 38.39,35.36 37.32,35.36 33.38,31.41 ATSAM3S4BA.24 32.76,30.79 32.76,29.72 34.28,28.2 34.28,27.4 | C10.2 39.42,25.6 38.38,26.64 37.62,26.64 36.84,27.4 34.28,27.4 | ATSAM3S4BA.54 24.16,24.31 22.7,22.86 19.68,22.86 | ATSAM3S4BA.64 28.66,21.74 28.67,22.71 30.34,24.38 31.88,24.38 | C18.2 18.59,22.5 18.95,22.86 19.68,22.86 | C7.1 C6.1 37.97,16.87 37.19,17.65 v37.19,18.84 36.81,19.22 36.81,19.47 35.48,20.8 34.98,21.28 ATSAM3S4BA.8 32.38,23.87 32.38,23.88 31.88,24.38 | 34.4,24.68 ATSAM3S4BA.12 33.46,25.63 32.51,25.63 | 27.11,20.19 27.11,18.61 27.69,18.03 27.69,15.89 v27.71,15.87 | 27.71,15.72 27.71,13.97 C9.2 | 19.68,22.86 20.19,22.35 20.19,21.84 v20.27,21.77 | 31.88,24.38 31.88,24.99 32.51,25.63 | 34.28,27.4 32.51,25.63
  Bottom 0.254: JP1.2 52.12,26.84 50.52,25.25 46.56,25.25 40.16,18.84 v37.19,18.84 | JTAG.1 4.78,17.68 6.45,16 | 6.45,16 7.37,15.09 8.18,15.09 11.56,15.11 14.07,17.63 16.13,17.63 16.54,18.03 21.08,18.03 | JTAG.2 2.24,16.81 3.05,16 6.45,16 | v27.7,15.88 v27.71,15.87 | SWITCH1.PIN1 22.77,7.66 23.18,7.66 26.2,10.68 26.2,13.71 27.7,15.22 v27.71,15.87 | v27.71,15.87 27.71,15.92 26.4,17.23 21.87,17.23 21.08,18.03 | v20.27,21.77 20.27,18.85 21.08,18.03
VX  (via drill 0.8 pad 1.02)
  Top 0.406: 1N4001.C 59.24,18.71 LF33CV.IN
  Bottom 0.406: LF33CV.IN 59.21,18.69 C1.1 58.98,22.01 58.98,22.06 59.13,22.2 59.13,23.49 59.92,24.28 63.45,24.28 v63.92,24.76 v63.93,24.76 63.93,26.49 1N1.C

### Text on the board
Top: PA2 | TST | PA0 | PA1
